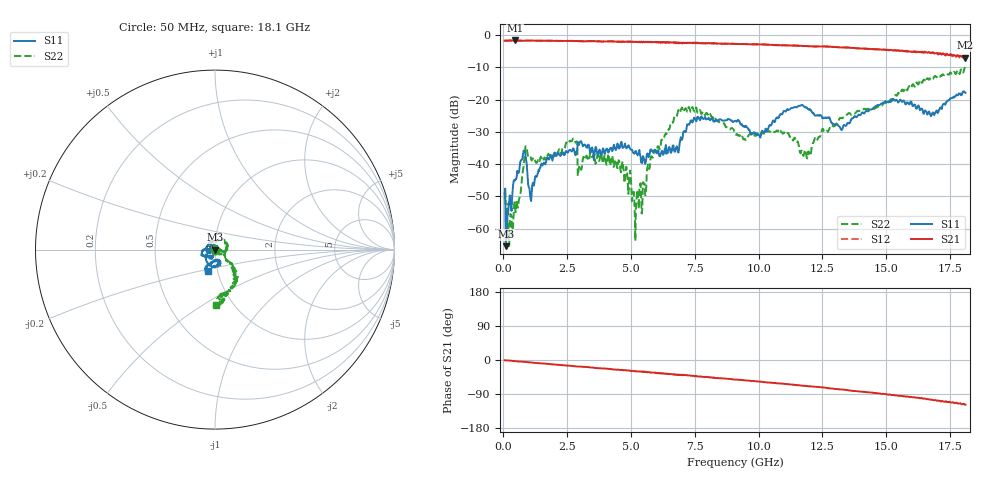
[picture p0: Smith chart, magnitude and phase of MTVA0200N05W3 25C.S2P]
! Network Analyzer HP8720D.06.14 Serial No. US36140669
! 17 Jan 2005  13:43:04
! Frequency  S11  S21  S12  S22
# HZ  S  DB R 50
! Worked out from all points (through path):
!   801 points, 50 MHz to 18.1 GHz, reference 50 ohm
!   highest |S21| = -1.71 dB at 456.1 MHz (marker M1); lowest = -7.0 dB at 18.1 GHz (marker M2)
!   group delay of S21, straight-line fit = 17.2 ps
!   lowest |S11| = -65.4 dB at 95.12 MHz (marker M3), VSWR 1.00, Z = 50 - j0.0317 ohm
!   |S11| at or under -10 dB: start of sweep to end of sweep
!   |S22| runs from -65.4 to -10.2 dB; largest |S21 - S12| = 0.026
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5e7  -49.29 -119.6  -1.76 -0.6  -1.78 -0.9  -51.05 -157.4
9.5125e7  -65.45 -36.4  -1.81 -0.8  -1.76 -1.3  -52.55 -48.0
2.75625e8  -52.43 104.8  -1.72 -1.9  -1.74 -2.2  -55.48 -22.9
4.56125e8  -45.11 85.3  -1.71 -2.8  -1.73 -3.2  -52.05 5.9
7.72e8  -36.89 57.7  -1.79 -4.7  -1.78 -4.9  -41.73 -80.7
9.299375e8  -41.47 -16.4  -1.75 -5.5  -1.76 -5.8  -35.75 167.0
1.110438e9  -48.98 78.8  -1.75 -6.6  -1.70 -7.1  -38.89 127.0
1.787312e9  -38.59 71.9  -1.80 -10.7  -1.77 -10.8  -37.06 108.7
2.689812e9  -36.03 68.1  -1.82 -15.7  -1.84 -16.0  -32.81 107.3
3.073375e9  -33.48 76.4  -1.93 -17.9  -1.89 -18.1  -41.12 -152.1
4.607625e9  -33.35 65.6  -2.16 -25.8  -2.12 -26.2  -42.55 136.0
5.216812e9  -36.65 100.1  -2.16 -30.2  -2.17 -30.5  -51.38 120.1
6.074188e9  -35.76 -148.7  -2.33 -35.2  -2.31 -35.3  -34.53 118.3
7.066938e9  -29.82 143.2  -2.43 -40.1  -2.48 -40.3  -23.78 41.4
9.075e9  -26.66 -165.9  -2.80 -51.4  -2.78 -51.8  -30.47 -51.0
1.000006e10  -30.93 -156.9  -2.93 -56.9  -2.92 -57.1  -30.02 -43.8
1.10605e10  -23.75 -177.7  -3.24 -63.3  -3.25 -63.8  -30.74 -42.9
1.209838e10  -23.93 -141.7  -3.50 -70.1  -3.52 -70.4  -34.13 -1.2
1.32265e10  -29.25 -111.0  -3.83 -77.6  -3.82 -78.0  -25.74 -11.3
1.509919e10  -20.80 -104.6  -4.75 -91.5  -4.60 -92.1  -20.56 -43.2
1.681394e10  -24.02 -85.8  -5.49 -105.0  -5.29 -105.6  -13.58 -61.7
1.81e10  -17.90 -108.3  -7.03 -118.0  -6.73 -118.1  -10.23 -89.4
